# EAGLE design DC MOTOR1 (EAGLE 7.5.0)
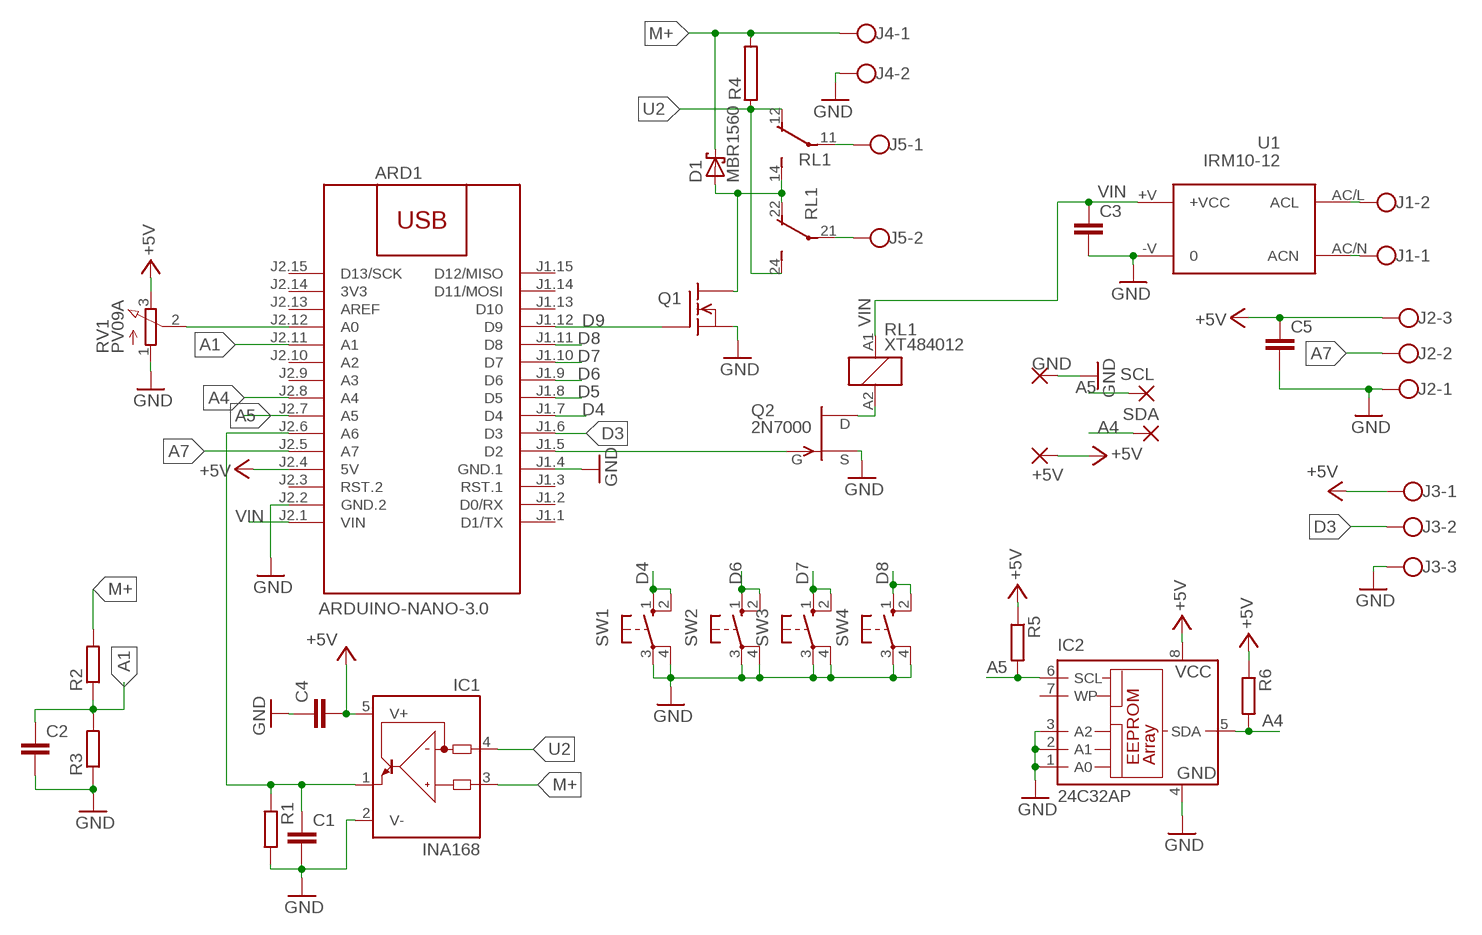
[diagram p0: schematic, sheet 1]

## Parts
+5V  2,15/1,0  [2,15/1,0]
ARD1  ARDUINO-NANO-3.0  [ARDUINO-NANO-3.0]
C1  C-EUC1206  [C1206]
C2  C-EUC1206  [C1206]
C3  C-EUC1206  [C1206]
C4  C-EUC1206  [C1206]
C5  C-EUC1206  [C1206]
D1  MBR1560  [TO220ACS]
GND  2,15/1,0  [2,15/1,0]
IC1  INA168  [SOT23-5]
IC2  24C32AP  [DIL8]
J1  W237-102  [W237-102]
J2  W237-103  [W237-103]
J3  W237-103  [W237-103]
J4  W237-102  [W237-102]
J5  W237-102  [W237-102]
Q1  MTP10N10EL  IRF840  [TO220]
Q2  2N7000  2N3819  [TO92]
R1  R-EU_R1206  [R1206]
R2  R-EU_R1206  [R1206]
R3  R-EU_R1206  [R1206]
R4  RAC07  [AC07]
R5  R-EU_R1206  [R1206]
R6  R-EU_R1206  [R1206]
RL1  XT484012  SR2Y5036  [SR2Y]
RV1  PV09A  [PTV09]
SCL  2,15/1,0  [2,15/1,0]
SDA  2,15/1,0  [2,15/1,0]
SW1  10-XX  [B3F-10XX]
SW2  10-XX  [B3F-10XX]
SW3  10-XX  [B3F-10XX]
SW4  10-XX  [B3F-10XX]
U1  IRM10-12  [IRM10-12]

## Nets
+5V: +5V.1(P) ARD1.J2.4(5V) C4.2 C5.1 IC1.5(V+) IC2.8(VCC) J2.3 J3.1 R5.1 R6.1 RV1.3(E)
A1: ARD1.J2.11(A1) C2.1 R2.1 R3.2
A4: ARD1.J2.8(A4) IC2.5(SDA) R6.2 SDA.1(P)
A5: ARD1.J2.7(A5) IC2.6(SCL) R5.2 SCL.1(P)
A7: ARD1.J2.5(A7) J2.2
D3: ARD1.J1.6(D3) J3.2
D4: ARD1.J1.7(D4) SW1.1(S) SW1.2(S1)
D5: ARD1.J1.8(D5)
D6: ARD1.J1.9(D6) SW2.1(S) SW2.2(S1)
D7: ARD1.J1.10(D7) SW3.1(S) SW3.2(S1)
D8: ARD1.J1.11(D8) SW4.1(S) SW4.2(S1)
D9: ARD1.J1.12(D9) Q1.1(G)
GND: ARD1.J1.4(GND.1) ARD1.J2.2(GND.2) C1.2 C2.2 C3.2 C4.1 C5.2 GND.1(P) IC1.2(V-) IC2.1(A0) IC2.2(A1) IC2.3(A2) IC2.4(GND) J2.1 J3.3 J4.2 Q1.3(S) Q2.3(S) R1.2 R3.1 RV1.1(A) SW1.3(P) SW1.4(P1) SW2.3(P) SW2.4(P1) SW3.3(P) SW3.4(P1) SW4.3(P) SW4.4(P1) U1.-V
M+: D1.C IC1.3(IN+) J4.1 R2.2 R4.2
N$1: ARD1.J2.6(A6) C1.1 IC1.1(OUT) R1.1
N$2: ARD1.J2.12(A0) RV1.2(S)
N$3: J1.1 U1.AC/N(ACN)
N$4: J1.2 U1.AC/L(ACL)
N$6: Q2.1(D) RL1.A2
N$7: J5.1 RL1.11(2:P)
N$8: J5.2 RL1.21(3:P)
N$9: ARD1.J1.5(D2) Q2.2(G)
N$12: D1.A Q1.2(D) RL1.14(2:S) RL1.22(3:O)
U2: IC1.4(IN-) R4.1 RL1.12(2:O) RL1.24(3:S)
VIN: ARD1.J2.1(VIN) C3.1 RL1.A1 U1.+V(+VCC)
Unconnected: ARD1.J1.1(D1/TX) ARD1.J1.2(D0/RX) ARD1.J1.3(RST.1) ARD1.J1.13(D10) ARD1.J1.14(D11/MOSI) ARD1.J1.15(D12/MISO) ARD1.J2.3(RST.2) ARD1.J2.9(A3) ARD1.J2.10(A2) ARD1.J2.13(AREF) ARD1.J2.15(D13/SCK) IC2.7(WP)

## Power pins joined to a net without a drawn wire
3V3: ARD1.J2.14(3V3)

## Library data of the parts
+5V GND SCL SDA = wirepad:2,15/1,0: THROUGH-HOLE PAD
ARD1 = diy-modules:ARDUINO-NANO-3.0: Arduino Nano 3.0 and compatible devices More details available here: https://www.arduino.cc/en/Main/ArduinoBoardNano Click here to find device on ebay.com
C1-C5 = rcl:C-EU: CAPACITOR, European symbol
D1 = diode:MBR1560
IC1 = burr-brown:INA168: High-Side Measurement Current Shunt Monitor; MF: TEXAS INSTRUMENTS; MPN: INA168NA/250; OC_FARNELL: 4375737; OC_NEWARK: 35C1744
IC2 = microchip:24*: Serial EEPROM I2C; MPN: AT24C32C-PU; OC_FARNELL: 1362652; OC_NEWARK: 50M3325
J1 J4 J5 = con-wago-500:W237-102: WAGO SCREW CLAMP; MPN: 237-102; OC_FARNELL: unknown; OC_NEWARK: 70K9898
J2 J3 = con-wago-500:W237-103: WAGO SCREW CLAMP; MPN: 237-103; OC_FARNELL: unknown; OC_NEWARK: 18M7116
Q1 = transistor-fet:IRF840: N-Channel Enhancement MOSFET (HEXFET); 500V; 8A; 0,85Ohm
Q2 = transistor-fet:2N3819: N-Channel Junction FET
R1-R3 R5 R6 = rcl:R-EU_: RESISTOR, European symbol
R4 = resistor-power:R: Power Resitor; OC_FARNELL: unknown; OC_NEWARK: unknown
RL1 = relay:SR2Y5*: Safety Relay 2 pole 6 A SCHRACK Source: http://www.schrack.com/.. 5809.pdf; OC_FARNELL: unknown; OC_NEWARK: unknown
RV1 = pot:PV09A
SW1-SW4 = switch-omron:10-XX: OMRON SWITCH; MPN: B3F-1000; OC_FARNELL: 176432; OC_NEWARK: 36M3542
U1 = acdc:IRM10-12

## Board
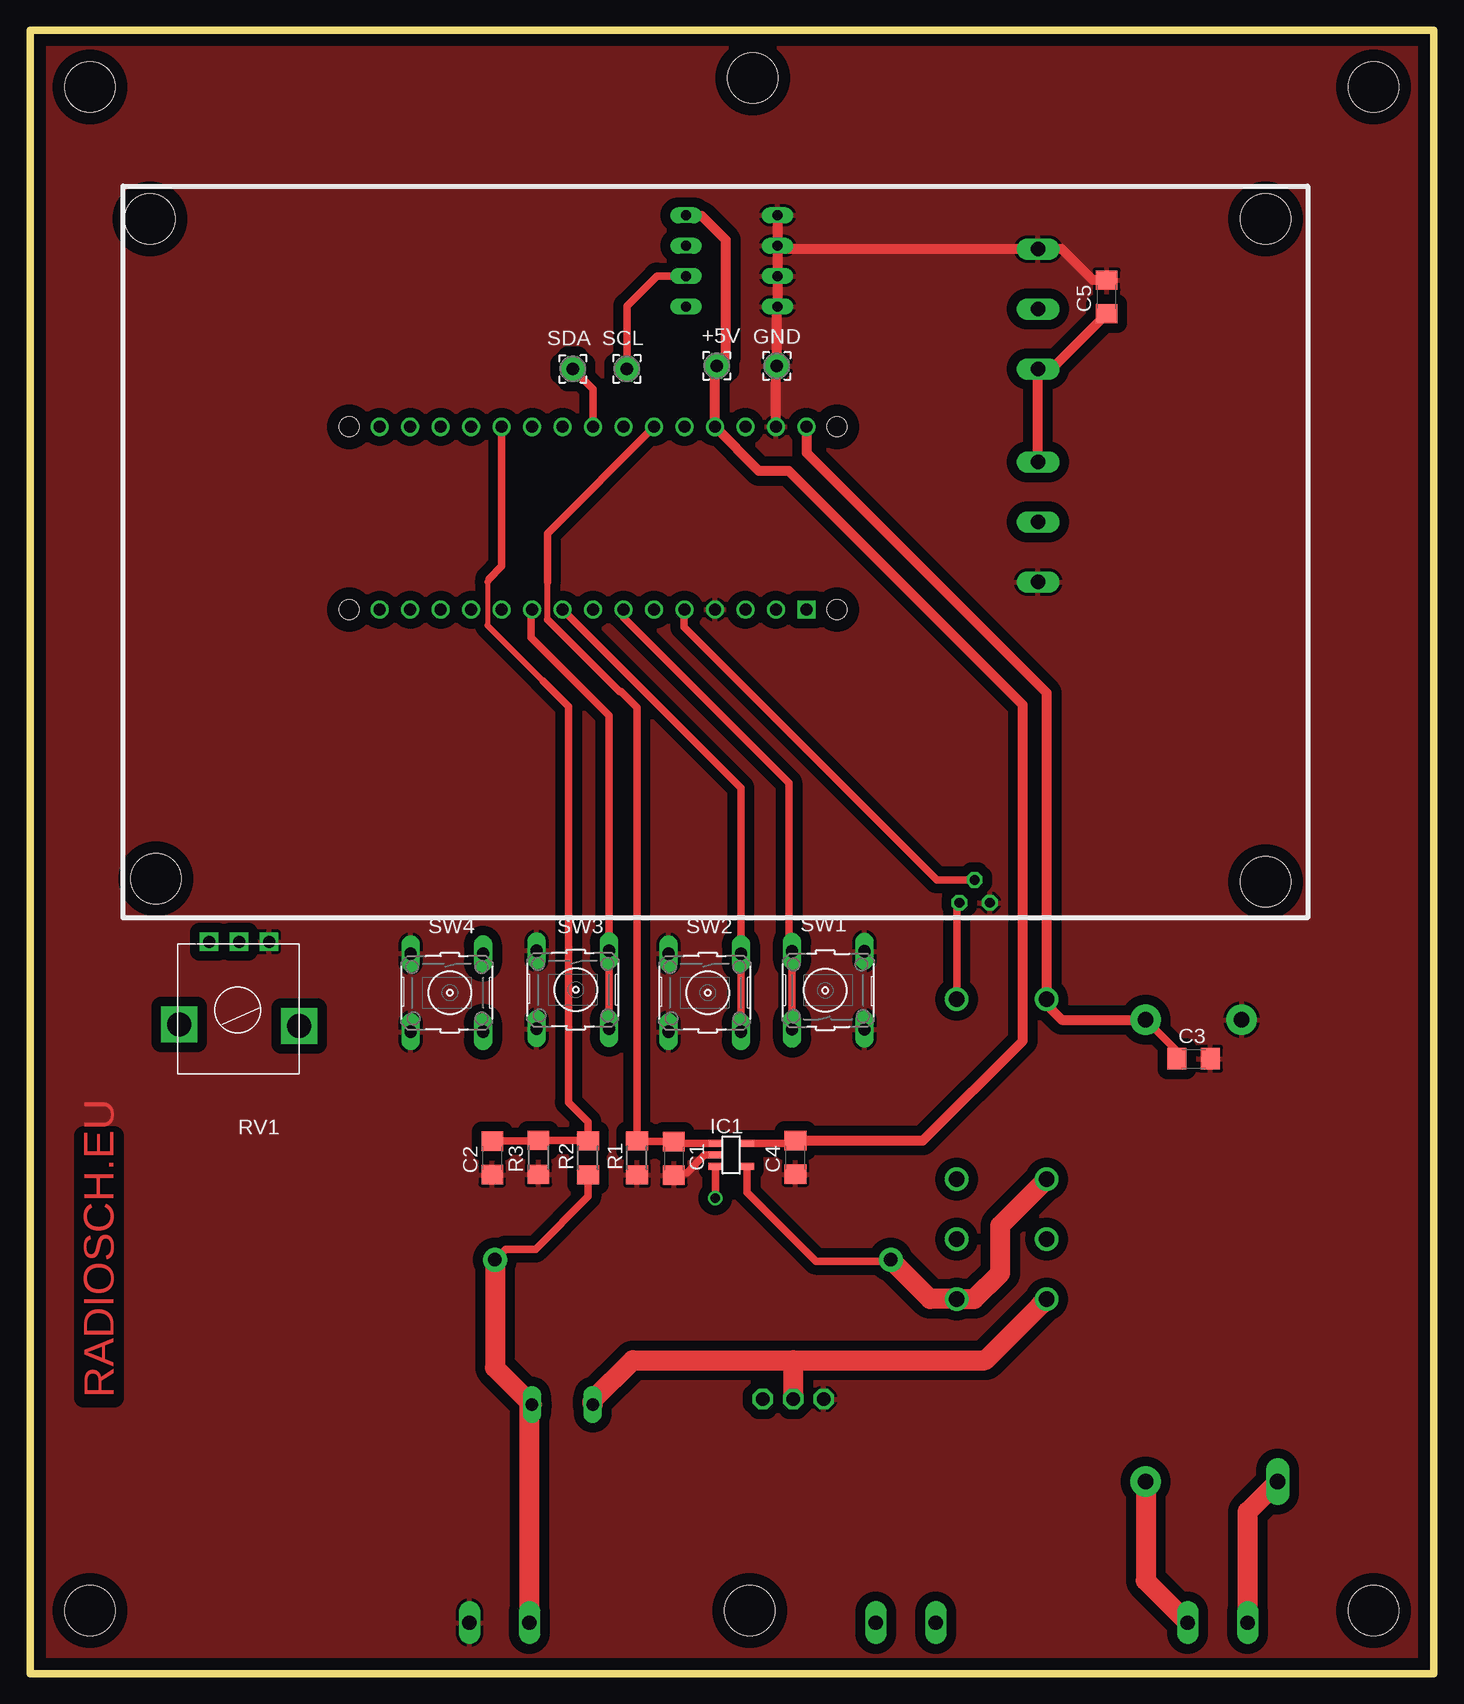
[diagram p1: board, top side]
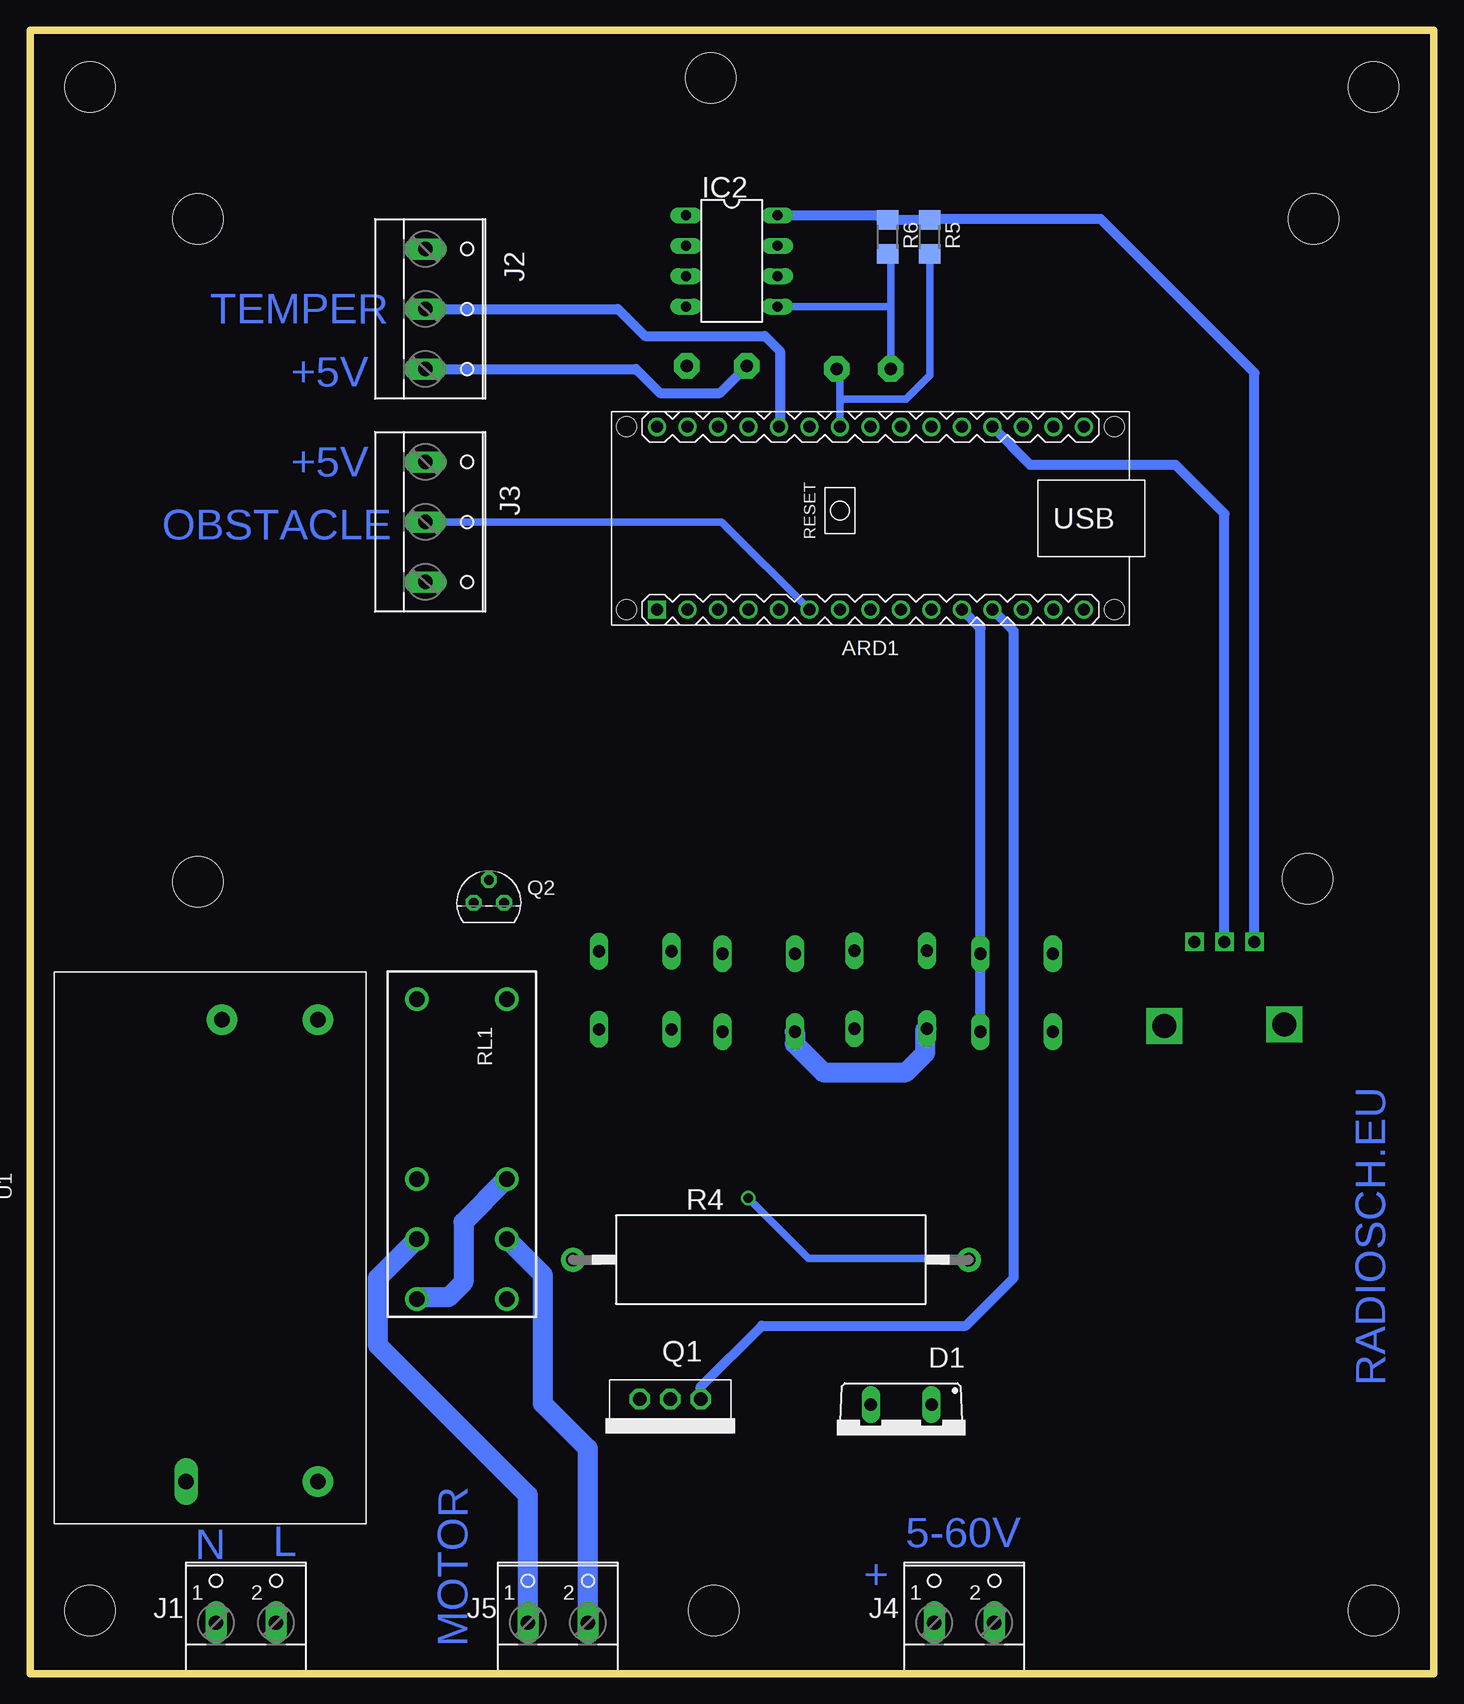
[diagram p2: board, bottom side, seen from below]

Size 117 x 137 mm. Coordinates in mm from the lower left corner, seen from the top.
Outline: 0,0 117,0 117,137 0,137 0,0
Copper layers (1*16): Top 0.035mm / dielectric 1.5mm / Bottom 0.035mm
Design rules "default": minimum track width 10mil, minimum drill 24mil, track to track 8mil, track to pad 8mil, pad to pad 8mil, via to via 8mil, smd to smd 8mil, copper to edge 40mil, drill to drill 8mil, minimum pad ring 10mil, minimum via ring 8mil, stop-mask expansion 4mil, vias tented up to drill 0mil, thermal gap 10mil
Holes 4.2 mm at 10,121.25 103,121.25 10.5,66.25 103,66 5,132.25 112,132.25 5,5.25 112,5.25 60,5.25 60.25,133

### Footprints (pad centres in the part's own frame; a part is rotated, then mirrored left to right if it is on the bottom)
2,15/1,0 = drill 1.016 pad 2.159 octagon: 1 0,0
ARDUINO-NANO-3.0 = drill 1 square: J1.1 17.78,7.62 | drill 1: J1.2 15.24,7.62; J1.3 12.7,7.62; J1.4 10.16,7.62; J1.5 7.62,7.62; J1.6 5.08,7.62; J1.7 2.54,7.62; J1.8 0,7.62; J1.9 -2.54,7.62; J1.10 -5.08,7.62; J1.11 -7.62,7.62; J1.12 -10.16,7.62; J1.13 -12.7,7.62; J1.14 -15.24,7.62; J1.15 -17.78,7.62; J2.1 17.78,-7.62; J2.2 15.24,-7.62; J2.3 12.7,-7.62; J2.4 10.16,-7.62; J2.5 7.62,-7.62; J2.6 5.08,-7.62; J2.7 2.54,-7.62; J2.8 0,-7.62; J2.9 -2.54,-7.62; J2.10 -5.08,-7.62; J2.11 -7.62,-7.62; J2.12 -10.16,-7.62; J2.13 -12.7,-7.62; J2.14 -15.24,-7.62; J2.15 -17.78,-7.62 | hole 1.651: -20.32,7.62; -20.32,-7.62; 20.32,-7.62; 20.32,7.62
C1206 = smd 1.6 x 1.8: 1 -1.4,0; 2 1.4,0
TO220ACS = drill 1.016 long: A 2.54,-2.54; C -2.54,-2.54
SOT23-5 = smd 0.6 x 1.2: 1 -0.95,-1.306; 2 0,-1.306; 3 0.95,-1.306; 4 0.95,1.306; 5 -0.95,1.306
DIL8 = drill 0.813 long: 1 -3.81,-3.81; 2 -1.27,-3.81; 3 1.27,-3.81; 4 3.81,-3.81; 5 3.81,3.81; 6 1.27,3.81; 7 -1.27,3.81; 8 -3.81,3.81
W237-102 = drill 1.194 long: 1 -2.5,-1.27; 2 2.5,-1.27
W237-103 = drill 1.194 long: 1 -5,-1.29; 2 0,-1.29; 3 5,-1.29
TO220 = drill 1.118 octagon: 1 -2.54,0; 2 0,0; 3 2.54,0
TO92 = drill 0.813 octagon: 1 1.27,0; 2 0,1.905; 3 -1.27,0
R1206 = smd 1.6 x 1.803: 1 -1.422,0; 2 1.422,0
AC07 = drill 1.1 pad 2: 1 -16.5,0; 2 16.5,0
SR2Y = drill 1.3: 11 7.54,-3.75; 12 2.54,-3.75; 14 12.54,-3.75; 21 7.54,3.75; 22 2.54,3.75; 24 12.54,3.75; A1 -12.46,-3.75; A2 -12.46,3.75
PTV09 = drill 1 square: 1 -2.5,0; 2 0,0; 3 2.5,0 | drill 2 square: P$4 -5,7; P$5 5,6.9
B3F-10XX = drill 1.016 long: 1 -3.251,2.761; 2 3.251,2.761; 3 -3.251,-3.261; 4 3.251,-3.261
IRM10-12 = drill 1.3 pad 2.54: +V 38.5,0; -V 38.5,8; AC/L 0,0 | drill 1.3 long: AC/N 0,11

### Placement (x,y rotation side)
+5V  57.25,109 0 top
ARD1  46.94,96.3 180 bottom
C1  53.67,42.94 270 top
C2  38.53,42.98 270 top
C3  97,51.25 0 top
C4  63.81,43.02 90 top
C5  89.75,114.75 90 top
D1  44.38,19.88 180 bottom
GND  62.25,109 90 top
IC1  58.45,43.23 270 top
IC2  58.5,117.75 270 bottom
J1  99,5.5 0 bottom
J2  82.75,113.75 270 bottom
J3  82.75,96 270 bottom
J4  39.12,5.5 0 bottom
J5  73,5.5 0 bottom
Q1  63.62,22.88 180 bottom
Q2  78.75,64.25 0 bottom
R1  50.6,42.98 270 top
R2  46.52,42.98 270 top
R3  42.39,43.02 90 top
R4  55.25,34.5 0 bottom
R5  42,119.75 270 bottom
R6  45.5,119.75 270 bottom
RL1  81,43.75 270 bottom
RV1  17.42,61 180 top
SCL  49.75,108.75 90 top
SDA  45.25,108.75 180 top
SW1  66.29,56.95 90 top
SW2  56.5,56.75 270 top
SW3  45.5,57 270 top
SW4  35,56.75 270 top
U1  93,16 90 bottom

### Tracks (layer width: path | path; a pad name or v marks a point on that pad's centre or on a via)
+5V
  Top 0.61: IC1.5 63.57,44.18 C4.2
  Top 0.813: IC2.8 54.75,121.5 56,121.5 58,119.5 58,109.75 +5V.1 57.1,108.85 ARD1.J2.4 60.77,100.25 63.25,100.25 82.75,80.75 82.75,52.75 74.42,44.42 C4.2 | C5.1 85.15,108.75 J2.3 J3.1
  Bottom 0.813: IC2.8 45.89,121.56 R6.1 R5.1 41.92,121.25 27.75,121.25 14.92,108.42 RV1.3 | J2.3 66.5,108.75 64.5,106.75 59.5,106.75 +5V.1
A1
  Top 0.406: 38.12,91 38.12,87.38
  Top 0.5: 38.25,91.25 38.25,91.12 38.12,91 | 38.12,87.38 42.75,82.75
  Top 0.61: ARD1.J2.11 39.32,92.32 38.25,91.25 | 42.75,82.75 44.88,80.62 44.88,47.62 46.5,46 46.5,44.42 R2.1 46.48,44.44 R3.2 42.33,44.38 C2.1
A4
  Top 0.61: ARD1.J2.8 46.94,107.06 SDA.1
  Bottom 0.61: SDA.1 45.25,114 | 45.25,114 45.25,118.08 R6.2 | IC2.5 45.31,113.94 45.25,114
A5
  Top 0.61: SCL.1 49.75,114 52.25,116.5 54.67,116.5 IC2.6
  Bottom 0.61: R5.2 42,108.25 44,106.25 49.23,106.25 49.48,106 | ARD1.J2.7 49.48,106 | 49.48,106 49.48,108.48 SCL.1
A7
  Bottom 0.813: J2.2 68,113.75 65.75,111.5 55.75,111.5 54.5,110.25 54.5,103.98 ARD1.J2.5
D3
  Bottom 0.61: J3.2 59.34,96 ARD1.J1.6
D4
  Top 0.61: ARD1.J1.7 49.48,88.02 63.25,74.25 63.25,60.48 SW1.2 SW1.1
D6
  Top 0.61: ARD1.J1.9 59.26,73.82 SW2.1 SW2.2
D7
  Top 0.61: SW3.2 SW3.1 48.26,79.86 41.75,86.38 41.75,88.57 ARD1.J1.10
D8
  Bottom 0.813: SW4.2 SW4.1 37.76,87.12 ARD1.J1.11
D9
  Bottom 0.813: Q1.1 61.09,23.91 56,29 39,29 35,33 35,86.9 ARD1.J1.12
GND
  Top 0.61: IC1.2 56.23,43.23 54.75,41.75 53.88,41.75 C1.2
  Top 0.813: IC2.2 62.58,118.75 J2.1 86,118.75 88.6,116.15 C5.2 | IC2.1 IC2.2 | IC2.2 IC2.3 IC2.4 62.25,113.88 GND.1 62.18,108.93 ARD1.J2.2
  Bottom 1.676: SW2.4 53.24,52.49 50.88,50.12 44,50.12 42.38,51.75 42.38,53.61 SW3.4
  pour Top (isolate 0.813): 1.25,135.75 116.25,135.75 116.25,1.25 1.25,1.25
M+  (via drill 0.8)
  Top 0.61: IC1.3 57.14,39.64 v57.12,39.62 | R2.2 46.52,39.77 42.12,35.38 39.62,35.38 R4.2
  Top 1.676: J4.1 41.62,22.2 D1.C 38.75,25.5 R4.2
  Bottom 0.61: v57.12,39.62 52.12,34.62 38.88,34.62 R4.2
N$1
  Top 0.5: 43.12,87.88 43.12,91
  Top 0.61: IC1.1 53.83,44.18 C1.1 50.66,44.34 R1.1 50.6,80.53 49.25,81.88 49.12,81.88 43.12,87.88 | 43.12,91 43.12,95.03 ARD1.J2.6
N$2
  Bottom 0.813: RV1.2 17.42,96.67 21.5,100.75 33.61,100.75 ARD1.J2.12
N$3
  Top 1.676: J1.1 101.5,13.5 U1.AC/N
N$4
  Top 1.676: U1.AC/L 93,7.73 J1.2
N$6
  Top 0.61: RL1.A2 77.25,64.02 Q2.1
N$7
  Bottom 1.676: J5.1 75.5,14.88 88,27.38 88,32.96 RL1.11
N$8
  Bottom 1.676: J5.2 70.5,18.75 74.25,22.5 74.25,33.21 RL1.21
N$9
  Top 0.61: Q2.2 75.59,66.16 54.5,87.25 54.5,88.62 ARD1.J1.5
N$12
  Top 1.676: D1.A 46.91,22.79 50.25,26.12 63.62,26.12 | 63.62,26.12 79.62,26.12 84.25,30.75 84.29,30.75 RL1.14 | Q1.2 63.62,26.12
  Bottom 1.676: RL1.22 77.29,41.21 80.88,37.62 80.88,32.62 82.12,31.38 84.58,31.38 RL1.14
U2
  Top 0.61: IC1.4 59.76,40.12 65.5,34.38 71.62,34.38 R4.1
  Top 1.676: R4.1 75.04,31.21 RL1.24 78.71,31.21 80.88,33.38 80.88,37.34 RL1.12
VIN
  Top 0.61: C3.1 95.6,51.9 U1.+V
  Top 0.813: U1.+V 86,54.5 84.75,55.75 RL1.A1 84.75,81.75 64.75,101.75 64.75,103.89 ARD1.J2.1

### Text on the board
Top: RADIOSCH.EU
Bottom: TEMPER | +5V | +5V | OBSTACLE | RADIOSCH.EU | 5-60V | L | N | + | MOTOR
